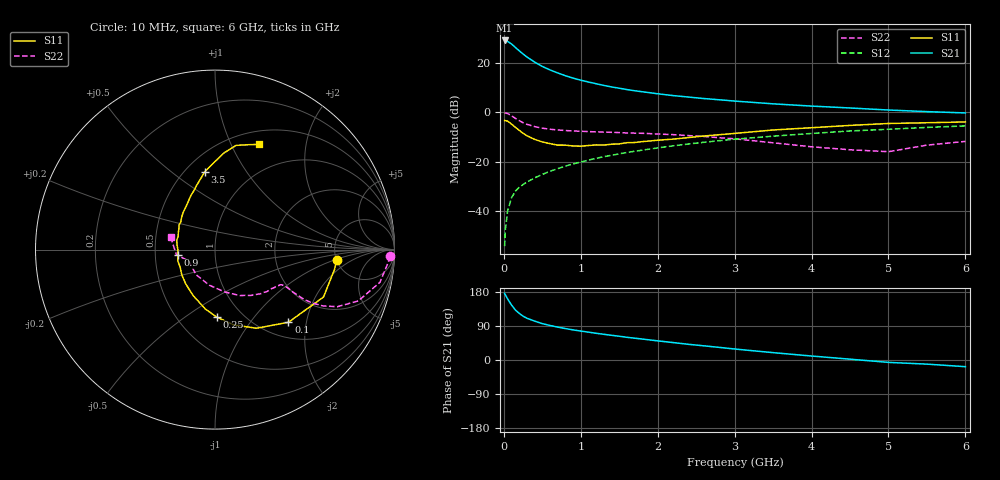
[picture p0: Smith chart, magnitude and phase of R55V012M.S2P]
! SIEMENS Small Signal Semiconductors
! BFR183
! Si NPN RF Bipolar Junction Transistor in SOT23
! VCE = 5 V  IC = 12 mA
! Common Emitter S-Parameters:  May  1996
# GHz  S  MA  R  50
!  f  S11  S21  S12  S22
! GHz  MAG  ANG  MAG  ANG  MAG  ANG  MAG  ANG
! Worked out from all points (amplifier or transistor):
!   36 points, 10 MHz to 6 GHz, reference 50 ohm
!   highest |S21| = 28.9 dB at 10 MHz (marker M1)
!   |S21| within 3 dB of that: start of sweep to 156.6 MHz
!   unconditionally stable (mu >= 1): 734.7 MHz to 2.504 GHz
!   at 250 MHz: K = 0.67, MSG = 26.3 dB, |S12| = -29.1 dB
!   at 1.4 GHz: K = 1.05, MAG = 12.4 dB, |S12| = -17.4 dB
!   at 6 GHz: K = 0.89, MSG = 2.6 dB, |S12| = -5.5 dB
!   S11 on the Smith chart (normalised r, x): 10 MHz: 5.02, -1.06; 100 MHz: 1.30, -1.58; 250 MHz: 0.77, -0.67; 900 MHz: 0.66, -0.04; 3.5 GHz: 0.62, +0.67; 6 GHz: 0.65, +1.29
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0.01  0.6803 -4.8  27.87 175.8  0.002 92.4  0.9769 -2.2
0.02  0.675 -9.4  27.6 171.8  0.0043 87.7  0.9658 -4.6
0.05  0.6597 -23.6  26.58 160.9  0.0104 79.3  0.9369 -11.2
0.1  0.5756 -44.7  23.68 145.0  0.0189 71.7  0.8481 -19.7
0.15  0.4954 -62.2  20.13 132.0  0.0256 67.3  0.7526 -25.0
0.2  0.4313 -76.3  17.27 123.0  0.0306 65.6  0.6769 -27.6
0.25  0.3754 -88.6  14.86 115.7  0.0349 64.5  0.6149 -28.8
0.3  0.3359 -99.1  12.94 110.2  0.0392 64.4  0.5703 -29.2
0.4  0.2841 -115.2  10.23 102.6  0.0474 65.4  0.5124 -28.8
0.5  0.2517 -130.2  8.357 96.0  0.0558 66.0  0.4763 -28.2
0.6  0.2326 -142.7  7.105 91.1  0.0645 66.8  0.4537 -27.7
0.7  0.217 -153.6  6.176 86.8  0.0727 67.3  0.4389 -27.5
0.9  0.209 -171.3  4.859 79.5  0.0909 66.9  0.4188 -27.9
1.1  0.2135 173.0  4.055 73.5  0.1083 66.5  0.407 -29.5
1.3  0.2179 160.4  3.46 67.8  0.1269 65.8  0.3962 -31.1
1.6  0.243 145.4  2.855 59.9  0.1542 63.6  0.3817 -34.8
2.2  0.2866 124.7  2.161 46.0  0.2098 58.4  0.3531 -44.2
3  0.3737 105.7  1.676 29.0  0.2857 49.6  0.2911 -61.7
3.5  0.438 97.4  1.473 19.4  0.3288 43.3  0.2419 -77.1
4.5  0.5416 84.6  1.216 2.2  0.4187 31.0  0.1751 -126.7
5.5  0.613 72.4  1.027 -10.9  0.4936 19.4  0.217 -172.5
6  0.6361 67.2  0.966 -17.6  0.5295 11.8  0.2581 163.8
